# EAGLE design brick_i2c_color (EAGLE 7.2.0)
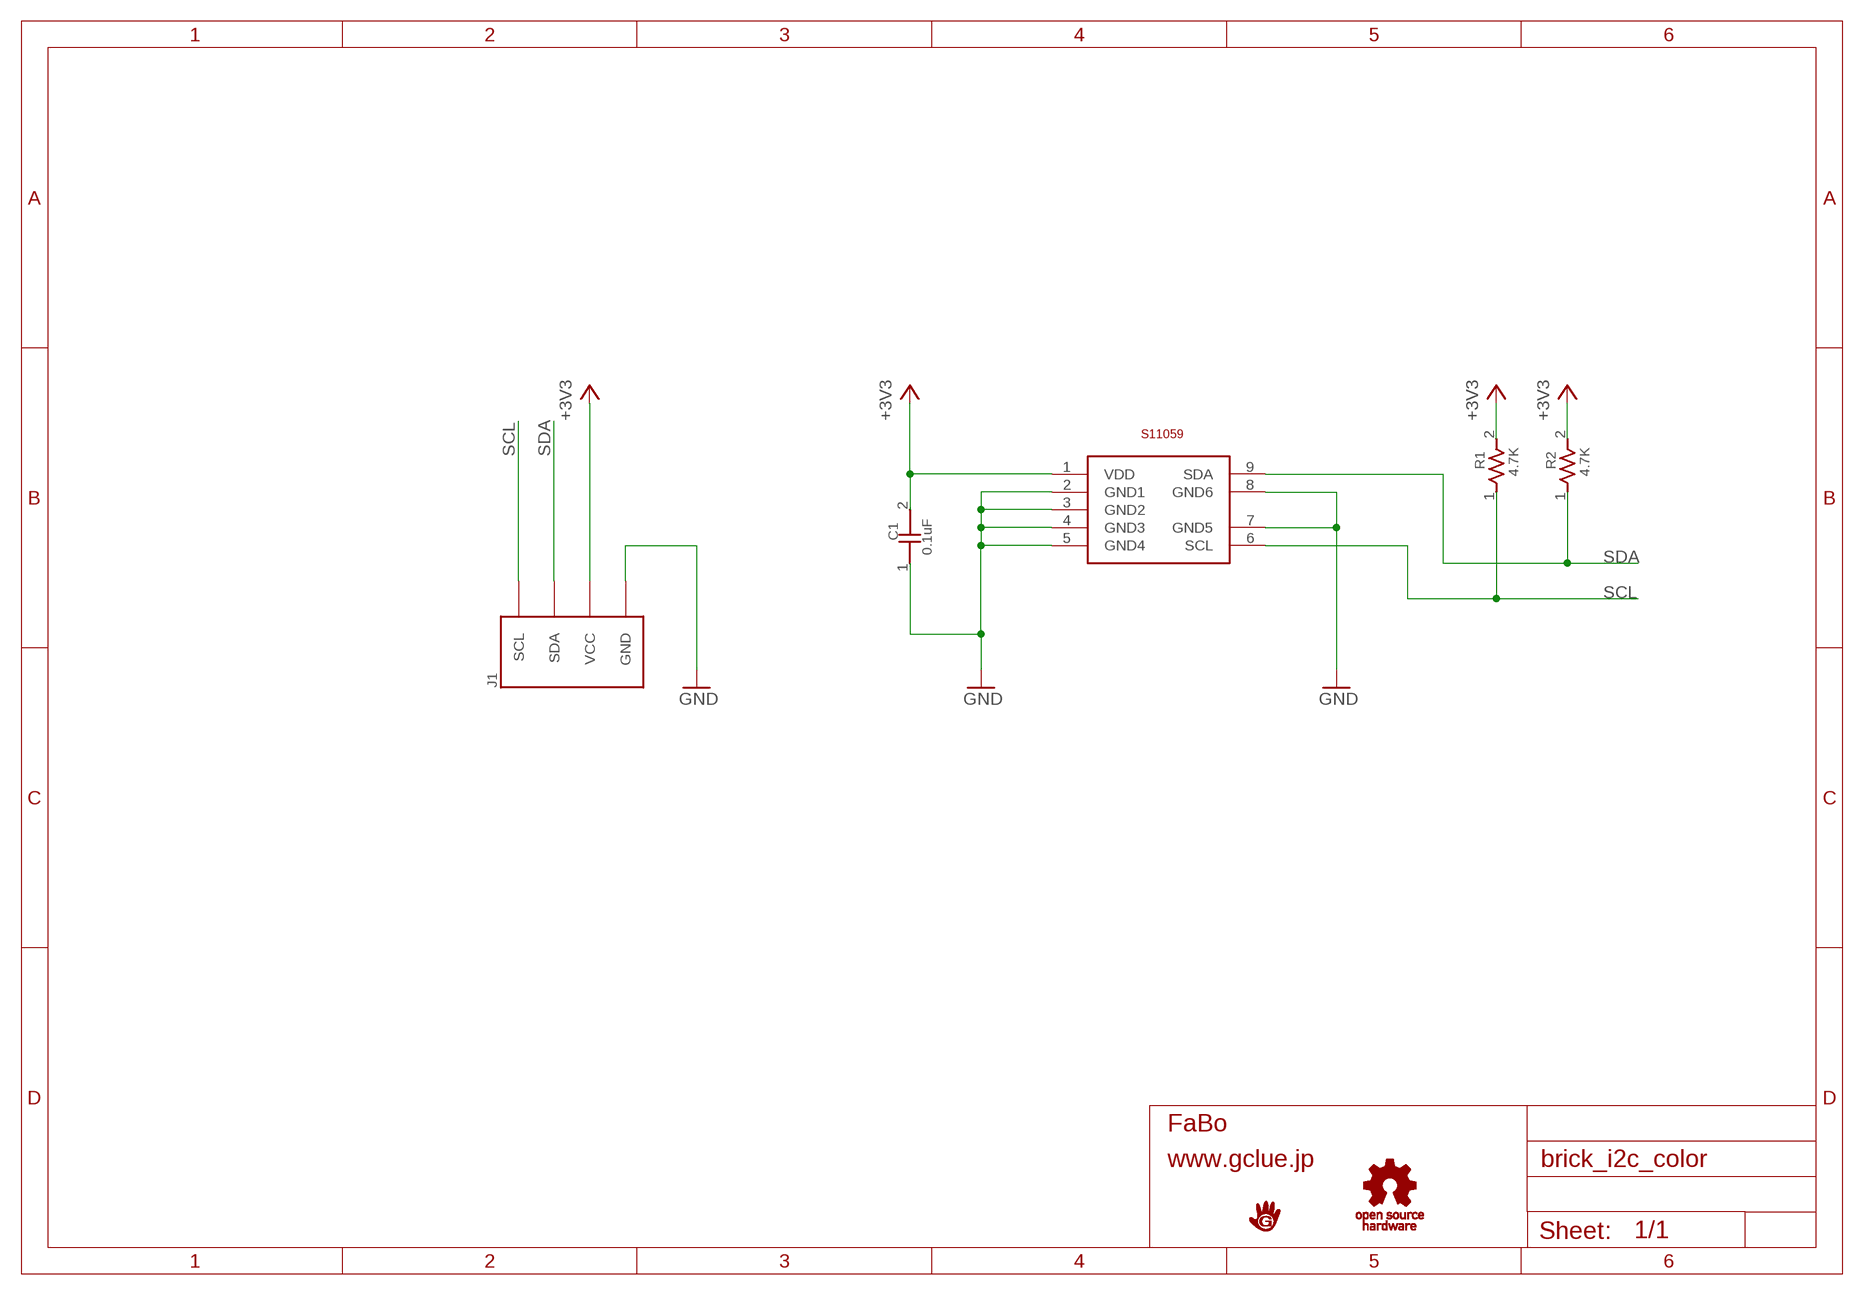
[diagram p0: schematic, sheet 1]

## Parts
C1  0.1uF  CAPACITOR0603  [0603]
J1  BRICK_I2C  [BRICK_I2C]
R1  4.7K  RESISTOR0603  [0603]
R2  4.7K  RESISTOR0603  [0603]
S1  HAMAMATSU-S11059  [HAMAMATSU-S11059]
U$2  LOGO_GCLUE-M  [LOGO_GCLUE_M]
U$3  LOGO_OSHW_T-M  [LOGO_OSHW_T_M]

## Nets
+3V3: C1.2 J1.VCC R1.2 R2.2 S1.1(VDD)
GND: C1.1 J1.GND S1.2(GND1) S1.3(GND2) S1.4(GND3) S1.5(GND4) S1.7(GND5) S1.8(GND6)
SCL: J1.SCL R1.1 S1.6(SCL)
SDA: J1.SDA R2.1 S1.9(SDA)

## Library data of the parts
C1 = GClue-Capacitor:CAPACITOR
J1 = gclue:BRICK_I2C: FaBo Brick 4pin(I2C)
R1 R2 = GClue-Resistors:RESISTOR
S1 = gclueSensor:HAMAMATSU-S11059
U$2 = gclue:LOGO_GCLUE
U$3 = gclue:LOGO_OSHW_T

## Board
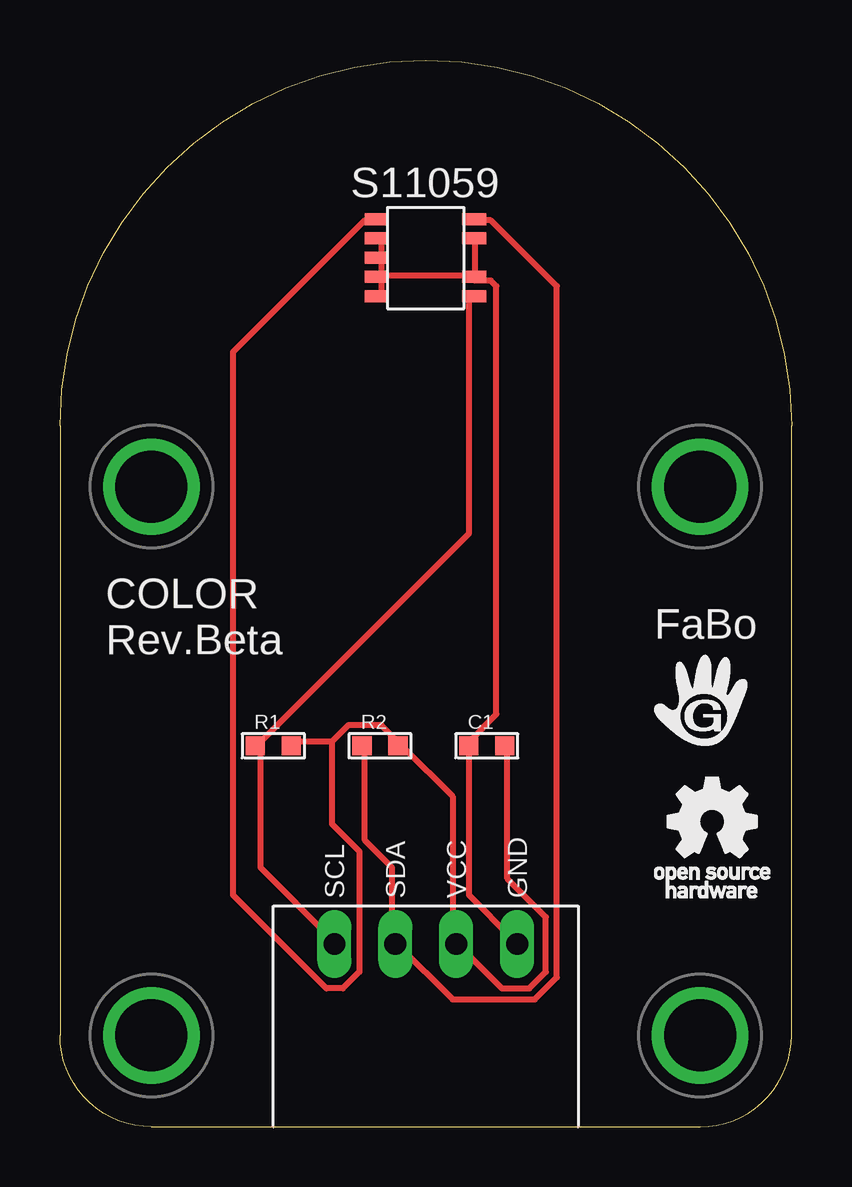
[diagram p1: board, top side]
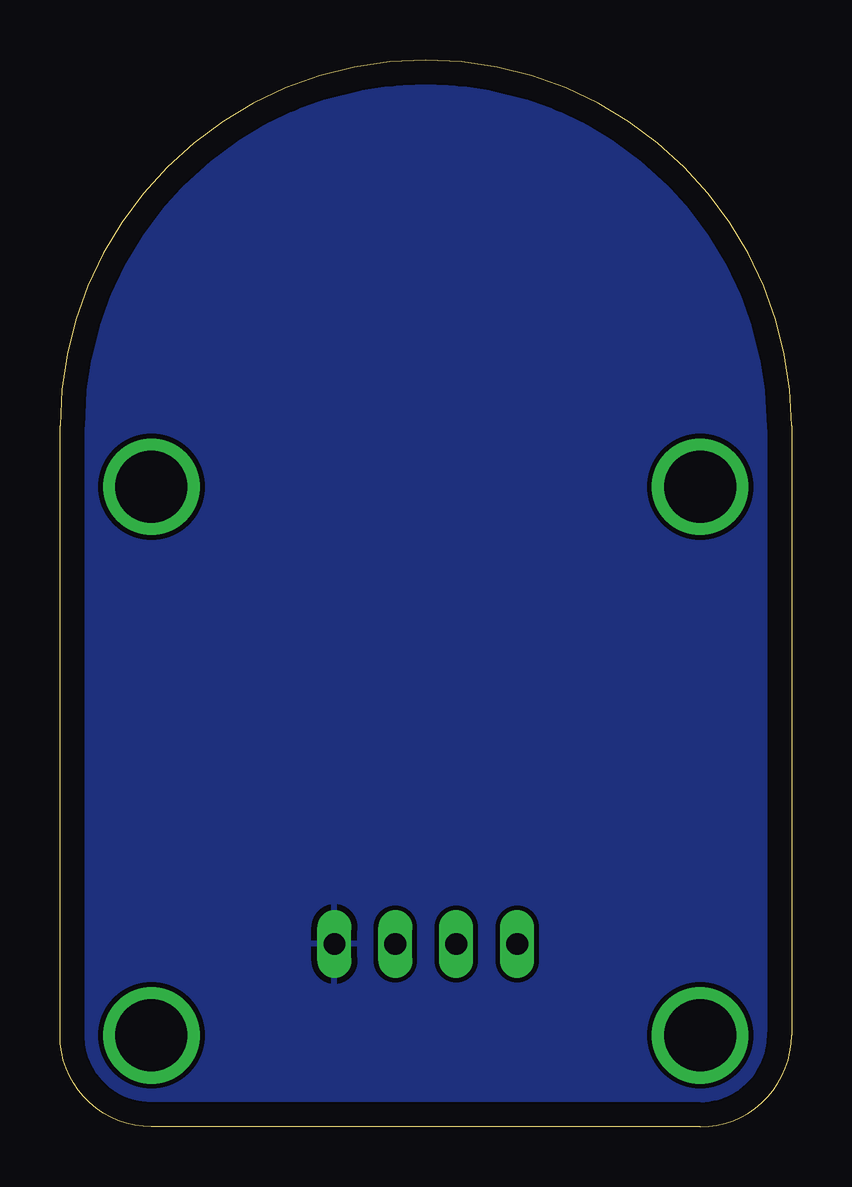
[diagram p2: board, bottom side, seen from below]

Size 30.48 x 44.45 mm. Coordinates in mm from the lower left corner, seen from the top.
Copper layers (1*16): Top 0.035mm / dielectric 1.5mm / Bottom 0.035mm
Design rules "default": minimum track width 10mil, minimum drill 24mil, track to track 8mil, track to pad 8mil, pad to pad 8mil, via to via 8mil, smd to smd 8mil, copper to edge 40mil, drill to drill 8mil, minimum pad ring 10mil, minimum via ring 8mil, stop-mask expansion 4mil, vias tented up to drill 0mil, thermal gap 10mil

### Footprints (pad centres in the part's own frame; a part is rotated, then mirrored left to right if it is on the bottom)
0603 = smd 0.8 x 0.8: 1 -0.75,0; 2 0.75,0
BRICK_I2C = drill 0.9 long: GND 3.81,-11.43; SCL -3.81,-11.43; SDA -1.27,-11.43; VCC 1.27,-11.43 | drill 3 pad 3.81: P$5 -11.43,7.62; P$6 11.43,7.62; P$7 -11.43,-15.24; P$8 11.43,-15.24
HAMAMATSU-S11059 = smd 1 x 0.5: 1 -2.04,1.62; 2 -2.04,0.82; 3 -2.04,0.02; 4 -2.04,-0.78; 5 -2.04,-1.58; 6 2.03,-1.58; 7 2.03,-0.78; 8 2.03,0.82; 9 2.03,1.62

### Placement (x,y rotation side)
C1  17.78,15.88 0 top
J1  15.24,19.05 0 top
R1  8.89,15.88 0 top
R2  13.33,15.88 0 top
S1  15.24,36.2 0 top
U$2  26.67,17.78 0 top
U$3  27.3,12.07 0 top

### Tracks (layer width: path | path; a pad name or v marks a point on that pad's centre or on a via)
+3V3
  Top 0.254: C1.2 18.64,15.82 18.64,10.34 20.24,8.74 20.24,6.45 19.56,5.77 18.41,5.77 16.59,7.6 J1.VCC 16.36,7.82 16.36,13.77 14.3,15.82 R2.2 14.07,16.05 13.39,16.74 12.01,16.74 11.33,16.05 | 11.33,16.05 9.73,16.05 R1.2 | 11.33,16.05 11.33,12.62 12.47,11.48 12.47,6.45 11.79,5.77 11.1,5.77 7.21,9.65 7.21,32.28 12.7,37.77 13.16,37.77 S1.1
GND
  Top 0.254: S1.7 17.27,35.48 17.27,36.86 S1.8 | S1.5 13.39,34.8 13.39,35.26 S1.4 13.39,35.48 | S1.2 13.39,36.86 13.39,36.4 S1.3 13.39,36.17 13.39,35.48 | 13.39,35.48 17.04,35.48 S1.7 | J1.GND 18.87,7.82 17.04,9.65 17.04,15.82 C1.1 17.04,16.05 18.19,17.2 18.19,35.03 17.96,35.26 17.27,35.26 S1.7
  pour Bottom: -0.64,44.45 31.11,44.45 31.11,0 0,-0.63
SCL
  Top 0.254: J1.SCL 11.33,7.82 8.36,10.8 8.36,15.82 R1.1 8.36,16.05 17.04,24.74 17.04,34.57 S1.6
SDA
  Top 0.254: R2.1 12.7,15.82 12.7,11.94 13.84,10.8 13.84,7.82 J1.SDA 14.07,7.6 16.36,5.31 19.79,5.31 20.7,6.22 20.7,35.03 17.96,37.77 17.27,37.77 S1.9

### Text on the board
tPlace: COLOR / Rev.Beta | FaBo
